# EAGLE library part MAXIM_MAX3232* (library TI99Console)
True RS-232 Transceivers 3.0V to 5.5V, Low-Power up to 1Mbps, Using Four 0.1µF External Capacitors Source: http://pdfserv.maxim-ic.com/en/ds/MAX3222-MAX3241.pdf
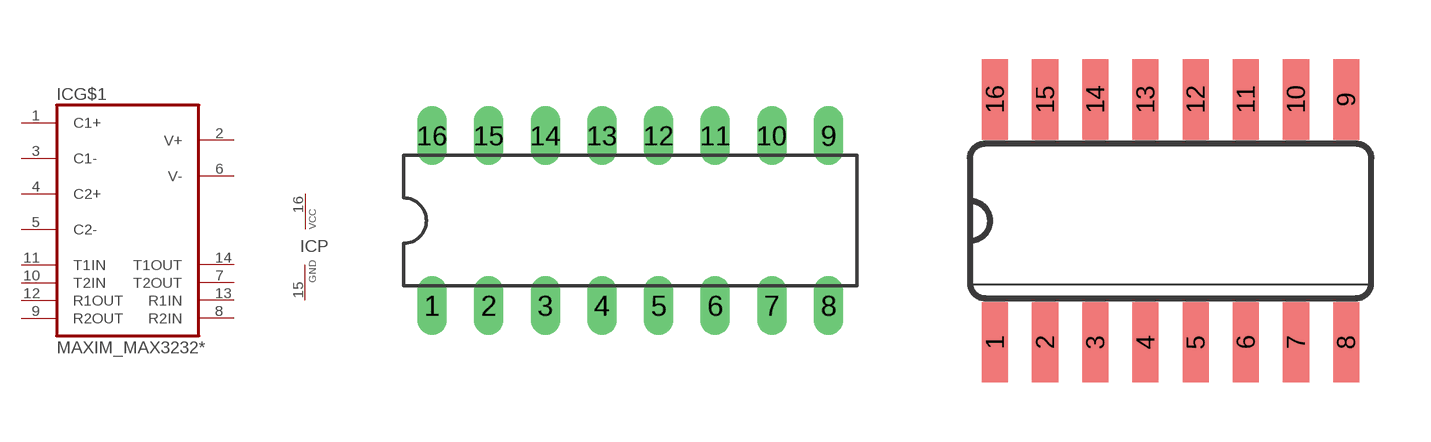
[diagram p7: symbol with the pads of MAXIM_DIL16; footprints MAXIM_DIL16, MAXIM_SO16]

Designator prefix IC; gates G$1=MAXIM_MAX232 P=MAXIM_VCC-GND

## MAXIM_MAX3232PE, MAXIM_MAX3232CPE (MF: MAXIM; MPN: MAX3232CPE+; OC_FARNELL: 9724494; OC_NEWARK: 68K4626), MAXIM_MAX3232EPE (MPN: MAX3232EPE+; OC_FARNELL: unknown; OC_NEWARK: 67K4860)  [MAXIM_DIL16]
1  G$1:C1+
2  G$1:V+
3  G$1:C1-
4  G$1:C2+
5  G$1:C2-
6  G$1:V-
7  G$1:T2OUT  out
8  G$1:R2IN  in
9  G$1:R2OUT  out
10  G$1:T2IN  in
11  G$1:T1IN  in
12  G$1:R1OUT  out
13  G$1:R1IN  in
14  G$1:T1OUT  out
15  P:GND  pwr
16  P:VCC  pwr

## MAXIM_MAX3232SE, MAXIM_MAX3232CSE (MPN: MAX3232CSE; OC_FARNELL: 9725490; OC_NEWARK: 90C2890), MAXIM_MAX3232ESE (MF: MAXIM; MPN: MAX3232ESE; OC_FARNELL: 9725539; OC_NEWARK: 79C3880)  [MAXIM_SO16]
Pads as for MAXIM_DIL16

## MAXIM_MAX3232UE, MAXIM_MAX3232CUE (MF: MAXIM; MPN: MAX3232CUE+; OC_FARNELL: 1593350; OC_NEWARK: 68K4629), MAXIM_MAX3232EUE (MF: MAXIM; MPN: MAX3232EUE+; OC_FARNELL: 1379769; OC_NEWARK: 68K4632)  [MAXIM_TSSOP16]
Pads as for MAXIM_DIL16

## MAXIM_MAX3232WE, MAXIM_MAX3232CWE (MF: MAXIM; MPN: MAX3232CWE+; OC_FARNELL: 9725504; OC_NEWARK: 68K4630), MAXIM_MAX3232EWE (MPN: MAX3232EWE+; OC_FARNELL: unknown; OC_NEWARK: 67K4863)  [MAXIM_SO16L]
Pads as for MAXIM_DIL16

## Footprint MAXIM_DIL16 (pad centres in mm)
Dual In Line Package
drill 0.813 long: 1 -8.89,-3.81; 2 -6.35,-3.81; 3 -3.81,-3.81; 4 -1.27,-3.81; 5 1.27,-3.81; 6 3.81,-3.81; 7 6.35,-3.81; 8 8.89,-3.81; 9 8.89,3.81; 10 6.35,3.81; 11 3.81,3.81; 12 1.27,3.81; 13 -1.27,3.81; 14 -3.81,3.81; 15 -6.35,3.81; 16 -8.89,3.81

## Footprint MAXIM_SO16 (pad centres in mm)
Small Outline Package .150 SIOC Source: http://www.maxim-ic.com/package_drawings/21-0041B.pdf
smd 0.66 x 2.032: 1 -4.445,-3.073; 2 -3.175,-3.073; 3 -1.905,-3.073; 4 -0.635,-3.073; 5 0.635,-3.073; 6 1.905,-3.073; 7 3.175,-3.073; 8 4.445,-3.073; 9 4.445,3.073; 10 3.175,3.073; 11 1.905,3.073; 12 0.635,3.073; 13 -0.635,3.073; 14 -1.905,3.073; 15 -3.175,3.073; 16 -4.445,3.073

## Footprint MAXIM_TSSOP16 (pad centres in mm)
Thin Shrink Small Outline Plastic 16 http://www.maxim-ic.com .. MAX3223-MAX3243.pdf
smd 0.305 x 0.991: 1 -2.275,-2.918; 2 -1.625,-2.918; 3 -0.975,-2.918; 4 -0.325,-2.918; 5 0.325,-2.918; 6 0.975,-2.918; 7 1.625,-2.918; 8 2.275,-2.918; 9 2.275,2.918; 10 1.625,2.918; 11 0.975,2.918; 12 0.325,2.918; 13 -0.325,2.918; 14 -0.975,2.918; 15 -1.625,2.918; 16 -2.275,2.918

## Footprint MAXIM_SO16L (pad centres in mm)
Small Outline Package .300 SIOC Source: http://www.maxim-ic.com/cgi-bin/packages?pkg=16%2FSOIC%2E300&Type=Max
smd 0.66 x 2.032: 1 -4.445,-4.902; 2 -3.175,-4.902; 3 -1.905,-4.902; 4 -0.635,-4.902; 5 0.635,-4.902; 6 1.905,-4.902; 7 3.175,-4.902; 8 4.445,-4.902; 9 4.445,4.902; 10 3.175,4.902; 11 1.905,4.902; 12 0.635,4.902; 13 -0.635,4.902; 14 -1.905,4.902; 15 -3.175,4.902; 16 -4.445,4.902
